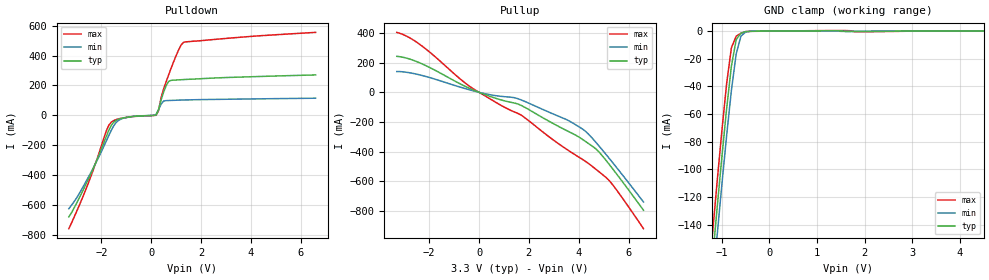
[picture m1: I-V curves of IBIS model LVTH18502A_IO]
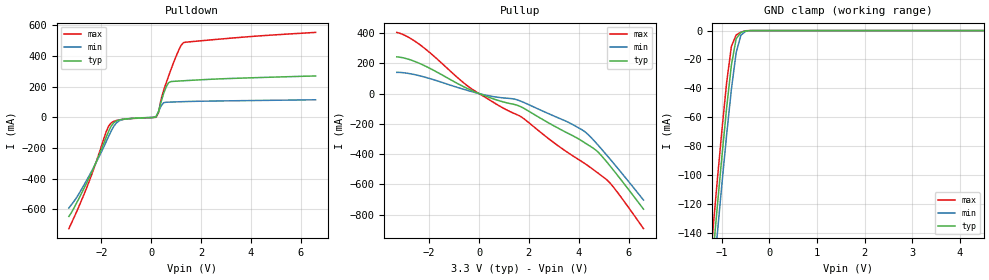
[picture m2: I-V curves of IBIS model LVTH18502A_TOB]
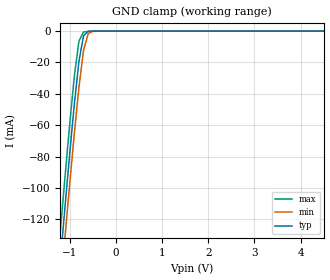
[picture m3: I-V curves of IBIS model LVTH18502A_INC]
|   TEXAS INSTRUMENTS INCORPORATED
|   Standard Linear and Logic
|   IBIS Model of SN74LVTH18502A
|   3.3V ABT SCAN TEST DEVICES WITH 18-BIT UNIVERSAL BUS TRANSCEIVERS
[IBIS Ver]   2.1
[Comment char]   |_char
[File Name]   sn74lvth18502a.ibs
[File Rev]   1.2   | from silicon model only
[Date]   01/31/2001
[Source]   Silicon-level SPICE model at Texas Instruments (ALEY)
[Notes]
   Release 1.0) 97104 ALEY
   Release 1.1) 97212 ALEY (based on process model updates)
   Release 1.2) 97215 ALEY - fixed load for ramp (rising) measurement
   includes all available commercial packages:
   PM=64TQFP (no-coupling model)
   - This file may be incomplete or may not be fully compliant
   with the IBIS specification. It will be replaced with a
   version that is IBIS Revision 3.2 compliant and is complete
   and accurate. Please email all questions and comments to
   sllibis@ti.com.
|   -For Questions or Comments please mailto:sllibis@ti.com
|  [Disclaimer]
|*   Property of Texas Instruments Incorporated.  Unauthorized   *
|*   reproduction and/or distribution is strictly prohibited.   *
|*   This product is protected under copyright law.   *
|*   Created 1995, (C) Copyright 1995, Texas Instruments Inc.,   *
|*   All Rights Reserved   *
|*   UNLESS THERE IS A SIGNED, WRITTEN AGREEMENT TO THE   *
|*   CONTRARY, TEXAS INSTRUMENTS ("TI") IS PROVIDING THE SPICE   *
|*   MODELS "AS IS" AND WITHOUT ANY WARRANTY, EXPRESSED OR   *
|*   IMPLIED.  TI assumes no liability for:   *
|*   1) the accuracy of the IBIS models provided to your   *
|*   company;   *
|*   2) the proper functioning of these IBIS models in your   *
|*   design or for any resulting applications; or   *
|*   3) infringement of patents, copyrights or intellectual   *
|*   property rights resulting from your use of these   *
|*   IBIS models.   *
|*   TI provides IBIS Models as a service to our customers.   *
|*   You and your company shall not distribute, sell or give   *
|*   these models to anyone else without prior written   *
|*   permission from TI.   *
|*   TI reserves the right to make changes to our products or   *
|*   to discontinue any semiconductor product or service   *
|*   without notice, and advises our customers to obtain the   *
|*   latest version of relevant information to verify, before   *
|*   placing orders, that the information being relied on is   *
|*   current.   *
|*   Please be aware that your receipt and use of the IBIS   *
|*   information provided shall serve as acceptance of these   *
|*   terms and conditions.  If you do not accept these terms,   *
|*   you should return or destroy the IBIS models and any   *
|*   other accompanying information immediately.   *
[Component]   SN74LVTH18502APM
[Manufacturer]  Texas Instruments
[Package]
|   typ   min   max
R_pkg   0.03   0.027   0.034
L_pkg   2.066nH   1.969nH   2.225nH
C_pkg   0.104pF   0.075pF   0.188pF
[Pin]   signal_name   model_name   R_pin   L_pin   C_pin
1   1A3   LVTH18502A_IO   0.03   2.212nH   0.188pF
2   1A4   LVTH18502A_IO   0.029   2.132nH   0.114pF
3   1A5   LVTH18502A_IO   0.03   2.093nH   0.099pF
4   GND   GND   0.03   2.08nH   0.106pF
5   1A6   LVTH18502A_IO   0.032   2.05nH   0.087pF
6   1A7   LVTH18502A_IO   0.032   2.015nH   0.08pF
7   1A8   LVTH18502A_IO   0.033   2.007nH   0.077pF
8   1A9   LVTH18502A_IO   0.032   1.99nH   0.08pF
9   VCC   POWER   0.033   2.074nH   0.09pF
10   2A1   LVTH18502A_IO   0.032   1.995nH   0.075pF
11   2A2   LVTH18502A_IO   0.032   2.025nH   0.08pF
12   2A3   LVTH18502A_IO   0.031   2.033nH   0.085pF
13   GND   GND   0.03   2.093nH   0.105pF
14   2A4   LVTH18502A_IO   0.031   2.142nH   0.1pF
15   2A5   LVTH18502A_IO   0.03   2.166nH   0.114pF
16   2A6   LVTH18502A_IO   0.029   2.225nH   0.188pF
17   2A7   LVTH18502A_IO   0.03   2.213nH   0.188pF
18   2A8   LVTH18502A_IO   0.031   2.161nH   0.114pF
19   2A9   LVTH18502A_IO   0.032   2.142nH   0.1pF
20   GND   GND   0.031   2.106nH   0.105pF
21   2NOEAB   LVTH18502A_INU   0.032   2.054nH   0.085pF
22   2LEAB   LVTH18502A_INC   0.032   2.017nH   0.077pF
23   2CLKAB   LVTH18502A_INC   0.033   2.065nH   0.079pF
24   TDI   LVTH18502A_INU   0.034   2.087nH   0.084pF
25   VCC   POWER   0.032   2.049nH   0.086pF
26   TCK   LVTH18502A_INT   0.032   1.989nH   0.075pF
27   2CLKBA   LVTH18502A_INC   0.032   2.014nH   0.079pF
28   2LEBA   LVTH18502A_INC   0.032   2.049nH   0.086pF
29   GND   GND   0.03   2.073nH   0.105pF
30   2NOEBA   LVTH18502A_INU   0.03   2.097nH   0.099pF
31   2B9   LVTH18502A_IO   0.031   2.142nH   0.114pF
32   2B8   LVTH18502A_IO   0.028   2.178nH   0.187pF
33   2B7   LVTH18502A_IO   0.028   2.167nH   0.187pF
34   2B6   LVTH18502A_IO   0.027   2.082nH   0.112pF
35   2B5   LVTH18502A_IO   0.029   2.08nH   0.099pF
36   GND   GND   0.029   2.064nH   0.105pF
37   2B4   LVTH18502A_IO   0.029   2.008nH   0.085pF
38   2B3   LVTH18502A_IO   0.03   1.98nH   0.079pF
39   2B2   LVTH18502A_IO   0.031   1.981nH   0.077pF
40   2B1   LVTH18502A_IO   0.031   1.976nH   0.08pF
41   VCC   POWER   0.033   2.005nH   0.081pF
42   1B9   LVTH18502A_IO   0.031   1.97nH   0.076pF
43   1B8   LVTH18502A_IO   0.031   1.996nH   0.08pF
44   1B7   LVTH18502A_IO   0.031   2.03nH   0.086pF
45   GND   GND   0.03   2.072nH   0.105pF
46   1B6   LVTH18502A_IO   0.03   2.102nH   0.1pF
47   1B5   LVTH18502A_IO   0.029   2.11nH   0.113pF
48   1B4   LVTH18502A_IO   0.028   2.155nH   0.186pF
49   1B3   LVTH18502A_IO   0.028   2.157nH   0.186pF
50   1B2   LVTH18502A_IO   0.028   2.09nH   0.112pF
51   1B1   LVTH18502A_IO   0.028   2.078nH   0.099pF
52   GND   GND   0.029   2.047nH   0.105pF
53   1NOEBA   LVTH18502A_IO   0.028   1.996nH   0.085pF
54   1LEBA   LVTH18502A_INC   0.029   1.969nH   0.079pF
55   1CLKBA   LVTH18502A_INC   0.031   1.97nH   0.077pF
56   TMS   LVTH18502A_INU   0.031   1.975nH   0.08pF
57   VCC   POWER   0.032   1.985nH   0.08pF
58   TDO   LVTH18502A_TOB   0.031   1.98nH   0.077pF
59   1CLKAB   LVTH18502A_INC   0.03   1.987nH   0.08pF
60   1LEAB   LVTH18502A_INC   0.03   2.022nH   0.086pF
61   GND   GND   0.029   2.068nH   0.105pF
62   1NOEAB   LVTH18502A_INU   0.03   2.086nH   0.099pF
63   1A1   LVTH18502A_IO   0.029   2.117nH   0.113pF
64   1A2   LVTH18502A_IO   0.029   2.167nH   0.186pF
| Models and submodels in the file (5): LVTH18502A_IO (I/O), LVTH18502A_TOB (3-state), LVTH18502A_INC (Input), LVTH18502A_INT (Input), LVTH18502A_INU (Input)
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[Model]   LVTH18502A_IO
| high-drive I/O buffer with bus-hold
| ibuf.lvta (97212 ALEY)
| tob.lvta  (97212 ALEY)
| pad.lvta  (97212 ALEY)
| Signals   1A1..1A9, 2A1..2A9, 1B1..1B9, 2B1..2B9
Model_type  I/O
Polarity   Non-Inverting
Enable   Active-Low
Vinl = 0.8V
Vinh = 2.0V
Vmeas= 1.5V
Cref = 50pf
Rref = 500
Vref = 0V
| variable   typ   min   max
C_comp   10p   NA   NA
[Temperature Range]   50   100   0
[Voltage range]   3.3   3   3.6
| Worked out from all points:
|   slope of the pulldown table from 0 to 0.495 V, typ, clamps not added: 3.25 ohm
|   slope of the pullup table from 0 to 0.495 V, typ, clamps not added: 16.2 ohm
|   GND clamp passes 1 mA (typ) near -0.56 V on its own axis
|Process range|   weak   strong
[pullup]
|   50C:3.3V:   100C:3V:weak   0C:3.6V:strong
|   Voltage   I(typ)   I(min)   I(max)
-3.3V     242.7mA    140.2mA    404.2mA
-2.8V     225.4mA    132.2mA    369.3mA
-2.3V     192.9mA    114.1mA    313.8mA
-300mV    20.86mA    13.18mA    31.49mA
700mV     -41.94mA   -23.2mA    -70.26mA
1.5V      -75.64mA   -39.93mA   -138.1mA
1.8V      -97.86mA   -58.74mA   -166.6mA
3.6V      -265.2mA   -191.6mA   -393.7mA
4.3V      -334.7mA   -267.1mA   -469.1mA
4.7V      -383.4mA   -339.3mA   -520.3mA
5.2V      -480.9mA   -440.4mA   -590.8mA
6.6V      -795.3mA   -739.8mA   -919.7mA
[pulldown]
|   50C:3.3V:   100C:3V:weak   0C:3.6V:strong
|   Voltage   I(typ)   I(min)   I(max)
-3.3V     -677.8mA   -623.8mA   -757mA
-2.5V     -420.1mA   -407.9mA   -444.4mA
-1.8V     -141.6mA   -172.1mA   -104.6mA
-1.6V     -67.02mA   -100.3mA   -45.51mA
-1.4V     -32.5mA    -46.74mA   -27.93mA
200mV     2.567mA    6.67mA     823.3uA
300mV     39.57mA    39.07mA    32.13mA
500mV     154.4mA    95.69mA    175mA
700mV     226.4mA    99.55mA    269.2mA
1.1V      237.5mA    101.9mA    436.1mA
1.3V      239.4mA    103mA      488.3mA
6.6V      270.5mA    114.9mA    554.8mA
[gnd_clamp]
|   50C:3.3V:   100C:3V:weak   0C:3.6V:strong
|   Voltage   I(typ)   I(min)   I(max)
-3.3V     -1.549A    -1.512A    -1.612A
-1.2V     -166.4mA   -186.3mA   -147.8mA
-1.1V     -128.1mA   -148mA     -109.1mA
-1V       -91.01mA   -111mA     -72.06mA
-900mV    -56mA      -75.56mA   -37.94mA
-800mV    -25.34mA   -42.9mA    -12mA
-700mV    -6.279mA   -16.54mA   -3.704mA
-600mV    -1.455mA   -3.641mA   -1.512mA
-500mV    -329uA     -657.6uA   -358.3uA
-300mV    -77.95uA   -53.31uA   -119.1uA
1.4V      233.8uA    101uA      404.8uA
6.6V      11.17nA    12.21nA    10.92nA
[ramp]
| variable   typ   min   max
dV/dt_r   1.5089E+00/4.8115E-10  1.1420E+00/1.4491E-09  1.7783E+00/2.2391E-10
dV/dt_f   1.7910E+00/8.5545E-10  1.6177E+00/2.2914E-09  1.9765E+00/4.1736E-10
[Model]   LVTH18502A_TOB
| three-state output buffer
| tob.lvta (97212 ALEY)
| pad.lvta (97212 ALEY)
| Signals   TDO
Model_type  3-state
Polarity   Non-Inverting
Enable   Active-Low
Vmeas= 1.5V
Cref = 50pf
Rref = 500
Vref = 0V
| variable   typ   min   max
C_comp   8p   NA   NA
[Temperature Range]   50   100   0
[Voltage range]   3.3   3   3.6
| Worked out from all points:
|   slope of the pulldown table from 0 to 0.495 V, typ, clamps not added: 3.25 ohm
|   slope of the pullup table from 0 to 0.495 V, typ, clamps not added: 16.2 ohm
|   GND clamp passes 1 mA (typ) near -0.58 V on its own axis
|Process range|   weak   strong
[pullup]
|   50C:3.3V:   100C:3V:weak   0C:3.6V:strong
|   Voltage   I(typ)   I(min)   I(max)
-3.3V     242.7mA    140.2mA    404.2mA
-2.8V     225.4mA    132.2mA    369.3mA
-2.3V     192.9mA    114.1mA    313.8mA
-300mV    20.86mA    13.18mA    31.49mA
700mV     -41.88mA   -23.15mA   -70.19mA
1.5V      -75.36mA   -39.76mA   -137.7mA
1.8V      -97.58mA   -58.87mA   -166.1mA
3.6V      -265.1mA   -191mA     -393.7mA
4.3V      -331mA     -259mA     -468.4mA
4.7V      -375mA     -326.3mA   -516.3mA
5.2V      -466.4mA   -421.4mA   -580.8mA
6.6V      -763.6mA   -703.5mA   -892.5mA
[pulldown]
|   50C:3.3V:   100C:3V:weak   0C:3.6V:strong
|   Voltage   I(typ)   I(min)   I(max)
-3.3V     -646.1mA   -591.2mA   -726.1mA
-2.5V     -398.2mA   -385.2mA   -423.3mA
-1.8V     -128.3mA   -158mA     -92.21mA
-1.6V     -56.18mA   -88.6mA    -35.51mA
-1.4V     -24.07mA   -37.43mA   -20.33mA
200mV     2.519mA    6.639mA    748.6uA
300mV     39.5mA     39.03mA    32.02mA
500mV     154.3mA    95.61mA    174.8mA
700mV     226.2mA    99.46mA    268.9mA
1.1V      237.3mA    101.8mA    435.7mA
1.3V      239.2mA    102.8mA    487.9mA
6.6V      270.5mA    114.9mA    554.8mA
[gnd_clamp]
|   50C:3.3V:   100C:3V:weak   0C:3.6V:strong
|   Voltage   I(typ)   I(min)   I(max)
-3.3V     -1.517A    -1.479A    -1.581A
-1.2V     -160.3mA   -179.4mA   -142.5mA
-1.1V     -123.2mA   -142.2mA   -105mA
-1V       -87.28mA   -106.4mA   -69.11mA
-900mV    -53.39mA   -72.1mA    -36.02mA
-800mV    -23.77mA   -40.53mA   -10.91mA
-700mV    -5.596mA   -15.18mA   -3.038mA
-600mV    -1.236mA   -3.105mA   -1.085mA
-500mV    -194.2uA   -518.2uA   -118.5uA
-400mV    -8.285uA   -43.13uA   -1.218uA
6.6V      7.886nA    8.661nA    7.714nA
[ramp]
| variable   typ   min   max
dV/dt_r   1.5081E+00/4.7366E-10  1.1387E+00/1.4512E-09  1.7781E+00/2.1597E-10
dV/dt_f   1.7910E+00/8.4858E-10  1.6182E+00/2.2837E-09  1.9768E+00/4.0623E-10
[Model]   LVTH18502A_INC
| high-impedance input buffer
| iclk.lvta (97212 ALEY)
| pad.lvta  (97212 ALEY)
| Signals   CLK, LE
Model_type  Input
Polarity   Non-Inverting
Vinl = 0.8V
Vinh = 2.0V
| variable   typ   min   max
C_comp   4p   NA   NA
[Temperature Range]   50   100   0
[Voltage range]   3.3   3   3.6
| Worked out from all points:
|   GND clamp passes 1 mA (typ) near -0.63 V on its own axis
|Process range|   weak   strong
[gnd_clamp]
|   50C:3.3V:   100C:3V:weak   0C:3.6V:strong
|   Voltage   I(typ)   I(min)   I(max)
-3.3V     -902.8mA   -920.5mA   -885.5mA
-1.2V     -145.7mA   -165.1mA   -126.6mA
-1.1V     -111.6mA   -131mA     -92.49mA
-1V       -78.36mA   -97.58mA   -59.49mA
-900mV    -46.84mA   -65.49mA   -29.02mA
-800mV    -19.33mA   -35.9mA    -6.331mA
-700mV    -3.025mA   -12.3mA    -602.9uA
-600mV    -177.8uA   -1.693mA   -229.1uA
-500mV    -5.2uA     -126.4uA   -50.31uA
6.6V      1.98nA     2.082nA    1.98nA
